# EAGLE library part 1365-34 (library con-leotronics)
DUAL ROW STRAIGHT HEADER 1364 SERIES. 1.27mm x 1.27mm. Without Fixing Post. SMT Source: http://www.leotronics.co.uk/Conexcon/Data%20Sheets/sec.%20A/1364ing.pdf
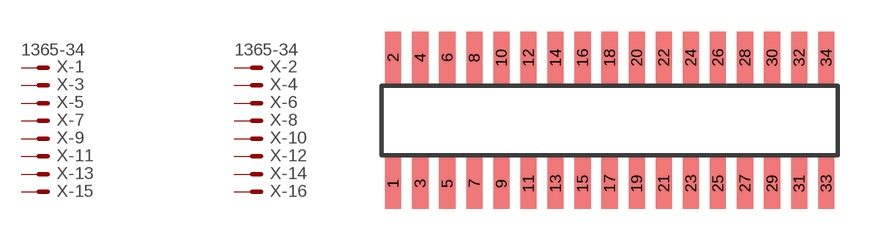
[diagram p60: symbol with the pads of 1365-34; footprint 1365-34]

Designator prefix X; gates -1=MVAL -2=MVAL -3=M -4=M -5=M -6=M -7=M -8=M -9=M -10=M -11=M -12=M -13=M -14=M -15=M -16=M -17=M -18=M -19=M -20=M -21=M -22=M -23=M -24=M -25=M -26=M -27=M -28=M -29=M -30=M -31=M -32=M -33=M -34=M

## 1365-34 (OC_FARNELL: unknown; OC_NEWARK: unknown)  [1365-34]
1  -1:S  pas
2  -2:S  pas
3  -3:S  pas
4  -4:S  pas
5  -5:S  pas
6  -6:S  pas
7  -7:S  pas
8  -8:S  pas
9  -9:S  pas
10  -10:S  pas
11  -11:S  pas
12  -12:S  pas
13  -13:S  pas
14  -14:S  pas
15  -15:S  pas
16  -16:S  pas
17  -17:S  pas
18  -18:S  pas
19  -19:S  pas
20  -20:S  pas
21  -21:S  pas
22  -22:S  pas
23  -23:S  pas
24  -24:S  pas
25  -25:S  pas
26  -26:S  pas
27  -27:S  pas
28  -28:S  pas
29  -29:S  pas
30  -30:S  pas
31  -31:S  pas
32  -32:S  pas
33  -33:S  pas
34  -34:S  pas

## Footprint 1365-34 (pad centres in mm)
DUAL ROW STRAIGHT HEADER 1364 SERIES. 1.27mm x 1.27mm. Without Fixing Post. SMT Source: http://www.leotronics.co.uk/Conexcon/Data%20Sheets/sec.%20A/1364ing.pdf
smd 0.76 x 2.4: 1 -10.16,-2.95; 2 -10.16,2.95; 3 -8.89,-2.95; 4 -8.89,2.95; 5 -7.62,-2.95; 6 -7.62,2.95; 7 -6.35,-2.95; 8 -6.35,2.95; 9 -5.08,-2.95; 10 -5.08,2.95; 11 -3.81,-2.95; 12 -3.81,2.95; 13 -2.54,-2.95; 14 -2.54,2.95; 15 -1.27,-2.95; 16 -1.27,2.95; 17 0,-2.95; 18 0,2.95; 19 1.27,-2.95; 20 1.27,2.95; 21 2.54,-2.95; 22 2.54,2.95; 23 3.81,-2.95; 24 3.81,2.95; 25 5.08,-2.95; 26 5.08,2.95; 27 6.35,-2.95; 28 6.35,2.95; 29 7.62,-2.95; 30 7.62,2.95; 31 8.89,-2.95; 32 8.89,2.95; 33 10.16,-2.95; 34 10.16,2.95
